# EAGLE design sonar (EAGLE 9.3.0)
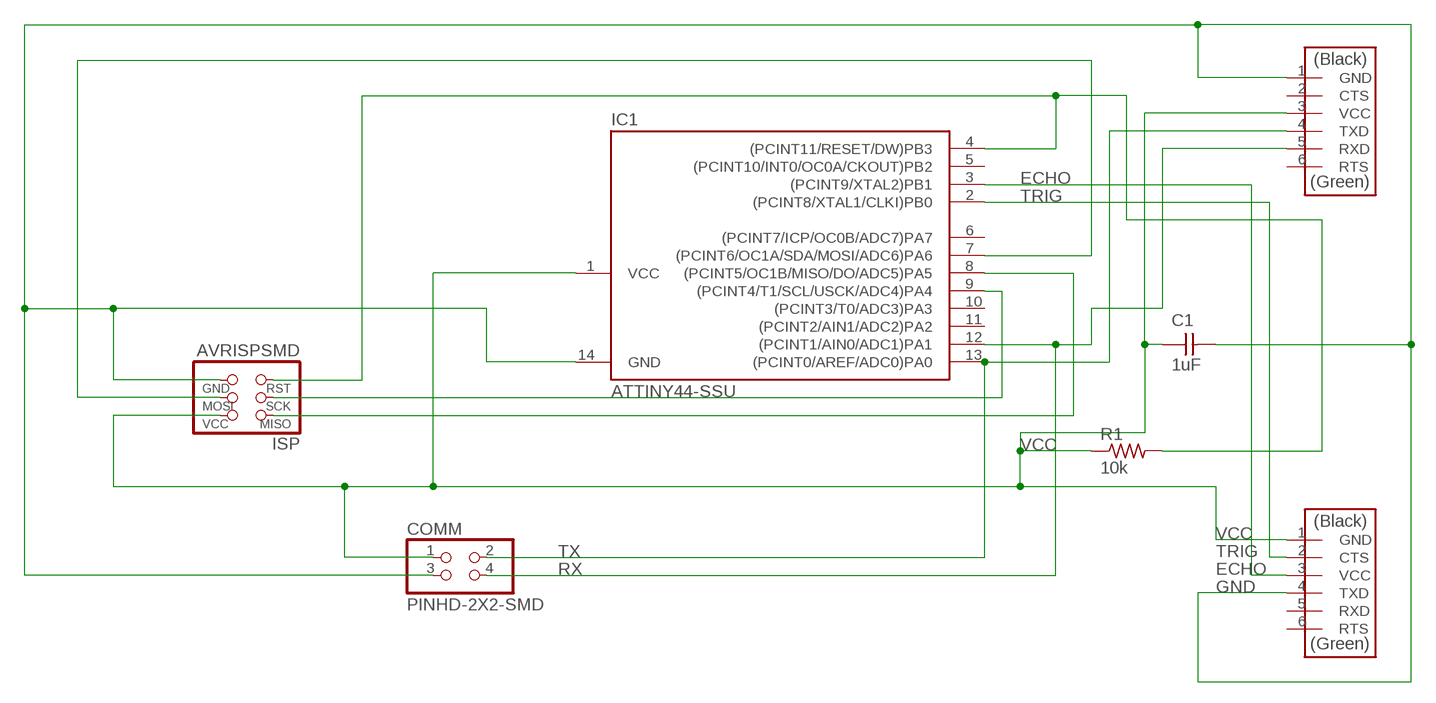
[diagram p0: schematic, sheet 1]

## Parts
C1  1uF  CAP-UNPOLARIZEDFAB  [C1206FAB]
COMM  PINHD-2X2-SMD  [2X02SMD]
FTDI  FTDI-SMD-HEADER  [1X06SMD]
IC1  ATTINY44-SSU  [SOIC14]
ISP  AVRISPSMD  [2X03SMD]
R1  10k  RES-US1206FAB  [R1206FAB]
SENSOR  FTDI-SMD-HEADER  [1X06SMD]

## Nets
ECHO: IC1.3((PCINT9/XTAL2)PB1) SENSOR.3(VCC)
GND: C1.2 COMM.3 FTDI.1(GND) IC1.14(GND) ISP.6(GND) SENSOR.4(TXD)
MISO: IC1.8((PCINT5/OC1B/MISO/DO/ADC5)PA5) ISP.1(MISO)
MOSI: IC1.7((PCINT6/OC1A/SDA/MOSI/ADC6)PA6) ISP.4(MOSI)
RST: IC1.4((PCINT11/RESET/DW)PB3) ISP.5(RST) R1.2
RX: COMM.4 FTDI.5(RXD) IC1.12((PCINT1/AIN0/ADC1)PA1)
SCK: IC1.9((PCINT4/T1/SCL/USCK/ADC4)PA4) ISP.3(SCK)
TRIG: IC1.2((PCINT8/XTAL1/CLKI)PB0) SENSOR.2(CTS)
TX: COMM.2 FTDI.4(TXD) IC1.13((PCINT0/AREF/ADC0)PA0)
VCC: C1.1 COMM.1 FTDI.3(VCC) IC1.1(VCC) ISP.2(VCC) R1.1 SENSOR.1(GND)
Unconnected: FTDI.2(CTS) FTDI.6(RTS) IC1.5((PCINT10/INT0/OC0A/CKOUT)PB2) IC1.6((PCINT7/ICP/OC0B/ADC7)PA7) IC1.10((PCINT3/T0/ADC3)PA3) IC1.11((PCINT2/AIN1/ADC2)PA2) SENSOR.5(RXD) SENSOR.6(RTS)

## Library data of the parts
C1 = fab:CAP-UNPOLARIZED
COMM = fab:PINHD-2X2-SMD
FTDI SENSOR = fab:FTDI-SMD-HEADER
IC1 = fab:ATTINY44
ISP = fab:AVRISP
R1 = fab:RES-US: Resistor (US Symbol)

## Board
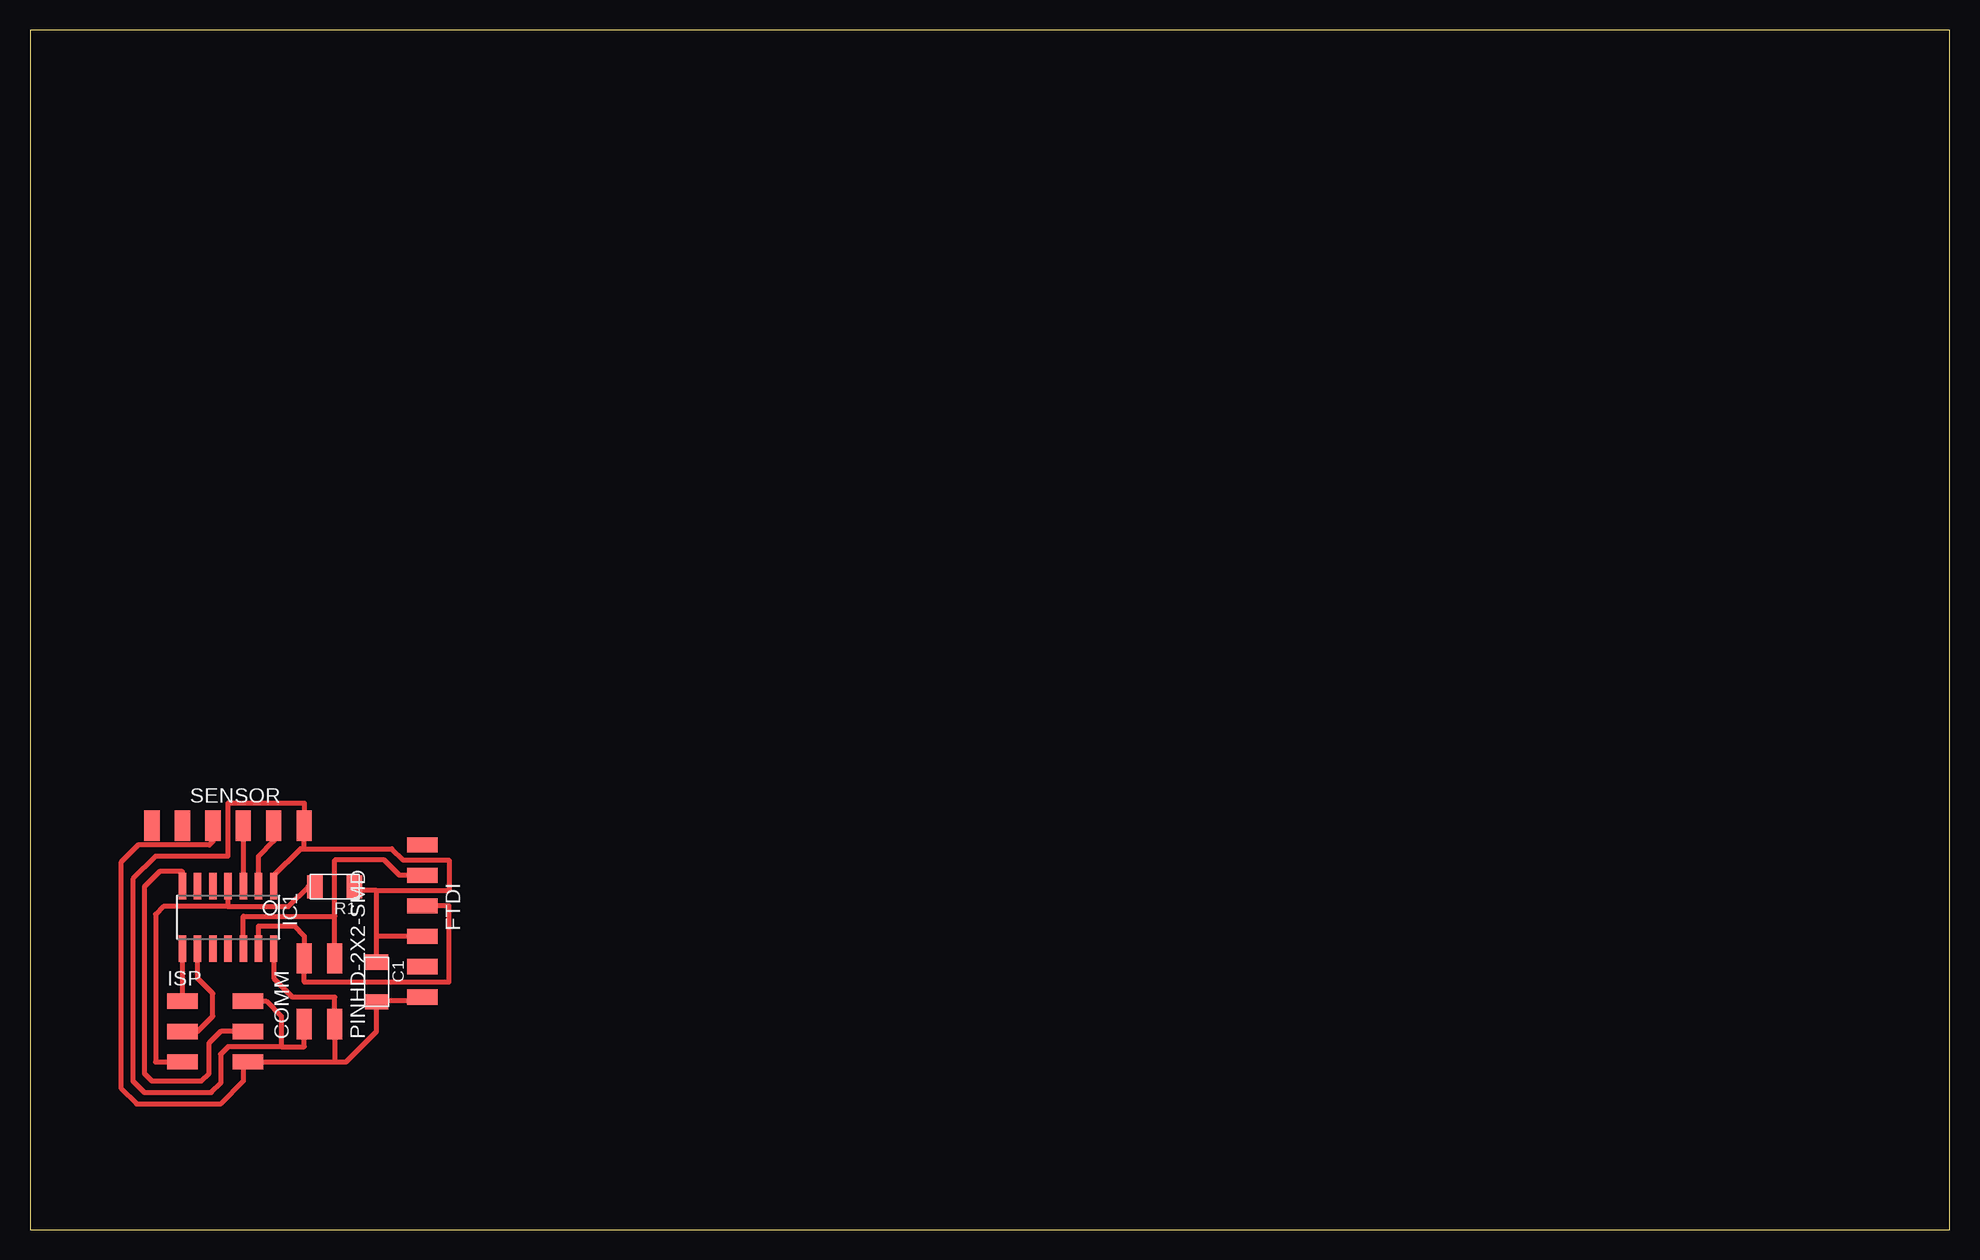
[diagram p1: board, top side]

Size 160 x 100 mm. Coordinates in mm from the lower left corner, seen from the top.
Outline: 0,0 160,0 160,100 0,100 0,0
Copper layers (1*16): Top 0.035mm / dielectric 1.5mm / Bottom 0.035mm
Design rules "eagle_fabcity-designrules *": minimum track width 16mil, minimum drill 32mil, track to track 16mil, track to pad 16mil, pad to pad 16mil, via to via 16mil, smd to smd 16mil, copper to edge 16mil, drill to drill 16mil, minimum pad ring 10mil, minimum via ring 8mil, stop-mask expansion 4mil, vias tented up to drill 0mil, thermal gap 16mil

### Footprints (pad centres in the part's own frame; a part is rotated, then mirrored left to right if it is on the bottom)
C1206FAB = smd 1.27 x 1.905: 1 -1.651,0; 2 1.651,0
2X02SMD = smd 2.54 x 1.27: 1 -2.54,1.27; 2 2.92,1.27; 3 -2.54,-1.27; 4 2.92,-1.27
1X06SMD = smd 2.54 x 1.27: 1 0,6.35; 2 0,3.81; 3 0,1.27; 4 0,-1.27; 5 0,-3.81; 6 0,-6.35
SOIC14 = smd 0.61 x 2.21: 1 -3.81,-2.603; 2 -2.54,-2.603; 3 -1.27,-2.603; 4 0,-2.603; 5 1.27,-2.603; 6 2.54,-2.603; 7 3.81,-2.603; 8 3.81,2.603; 9 2.54,2.603; 10 1.27,2.603; 11 0,2.603; 12 -1.27,2.603; 13 -2.54,2.603; 14 -3.81,2.603
2X03SMD = smd 2.54 x 1.27: 1 -2.54,2.54; 2 2.92,2.54; 3 -2.54,0; 4 2.92,0; 5 -2.54,-2.54; 6 2.92,-2.54
R1206FAB = smd 1.27 x 1.905: 1 -1.651,0; 2 1.651,0

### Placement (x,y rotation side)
C1  28.89,20.64 270 top
COMM  24.13,19.68 90 top
FTDI  32.7,25.72 180 top
IC1  16.51,26.04 180 top
ISP  15.24,16.51 0 top
R1  25.4,28.57 180 top
SENSOR  16.51,33.66 270 top

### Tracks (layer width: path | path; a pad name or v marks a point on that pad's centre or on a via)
ECHO
  Top 0.406: SENSOR.3 IC1.3
GND
  Top 0.406: 20.32,24.13 IC1.14 20.32,20.95 21.91,19.37 25.4,19.37 COMM.3 25.4,13.97 | FTDI.1 32.38,19.05 28.96,19.05 C1.2 28.89,16.51 26.35,13.97 25.4,13.97 | 25.4,13.97 ISP.6 17.78,13.97 17.78,12.38 15.88,10.48 8.89,10.48 7.62,11.75 7.62,30.66 9.01,32.04 14.95,32.04 15.24,32.33 SENSOR.4
MISO
  Top 0.406: IC1.8 ISP.1
MOSI
  Top 0.406: ISP.4 15.88,16.51 14.92,15.56 14.92,13.02 14.29,12.38 10.16,12.38 9.53,13.02 9.53,28.57 10.79,29.84 12.7,29.84 IC1.7
RST
  Top 0.406: ISP.5 10.48,13.97 10.48,26.29 11.11,26.92 16.51,26.92 | 23.43,28.57 R1.2 23.18,28.57 21.53,26.92 16.51,26.92 | 16.51,26.92 IC1.4
RX
  Top 0.406: 25.4,26.11 17.78,26.11 IC1.12 | 25.4,26.11 25.4,30.8 29.53,30.8 30.8,29.53 FTDI.5 | COMM.4 25.4,26.11
SCK
  Top 0.406: IC1.9 13.97,20.95 15.24,19.68 15.24,17.78 13.97,16.51 ISP.3
TRIG
  Top 0.406: IC1.2 19.05,31.11 20.32,32.38 SENSOR.2
TX
  Top 0.406: FTDI.4 34.92,26.99 34.92,20.64 34.29,20.64 22.86,20.64 COMM.2 22.86,24.45 22.01,25.3 19.05,25.3 IC1.13
VCC
  Top 0.406: 20.95,15.24 16.51,15.24 15.88,14.61 15.88,12.19 15.12,11.43 9.53,11.43 8.57,12.38 8.57,29.21 10.48,31.11 16.51,31.11 16.51,35.56 22.86,35.56 SENSOR.1 22.86,31.75 | ISP.2 19.68,19.05 20.95,17.78 20.95,15.24 | IC1.1 20.32,29.53 22.54,31.75 22.86,31.75 | 20.95,15.24 22.86,15.24 COMM.1 | 28.89,28.26 27.37,28.26 R1.1 | 32.38,24.13 FTDI.3 28.89,24.45 | C1.1 28.89,24.45 | 28.89,24.45 28.89,28.26 | 28.89,28.26 34.92,28.26 34.92,30.8 31.11,30.8 30.16,31.75 22.86,31.75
